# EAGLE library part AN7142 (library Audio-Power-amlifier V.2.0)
0,9W DUAL AUDIO POWER AMPLIFIER
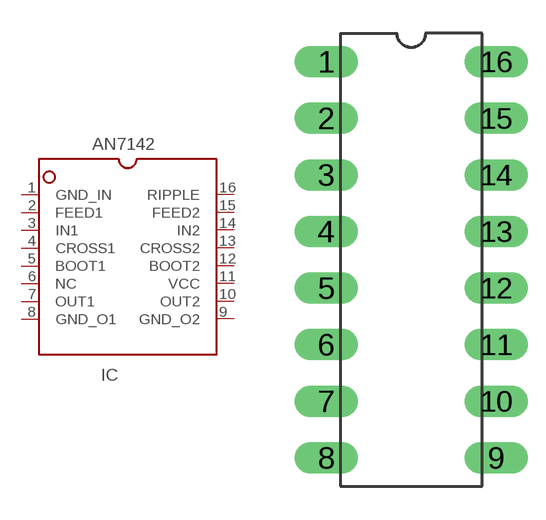
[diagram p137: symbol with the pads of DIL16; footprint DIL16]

Designator prefix IC

## AN7142  [DIL16]
1  GND_IN  pwr
2  FEED1
3  IN1  in
4  CROSS1
5  BOOT1
6  NC  nc
7  OUT1  out
8  GND_O1  pwr
9  GND_O2  pwr
10  OUT2  out
11  VCC  pwr
12  BOOT2
13  CROSS2
14  IN2  in
15  FEED2
16  RIPPLE

## Footprint DIL16 (pad centres in mm)
drill 0.8 pad 1.422 long: 1 -3.81,8.89; 2 -3.81,6.35; 3 -3.81,3.81; 4 -3.81,1.27; 5 -3.81,-1.27; 6 -3.81,-3.81; 7 -3.81,-6.35; 8 -3.81,-8.89; 9 3.81,-8.89; 10 3.81,-6.35; 11 3.81,-3.81; 12 3.81,-1.27; 13 3.81,1.27; 14 3.81,3.81; 15 3.81,6.35; 16 3.81,8.89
